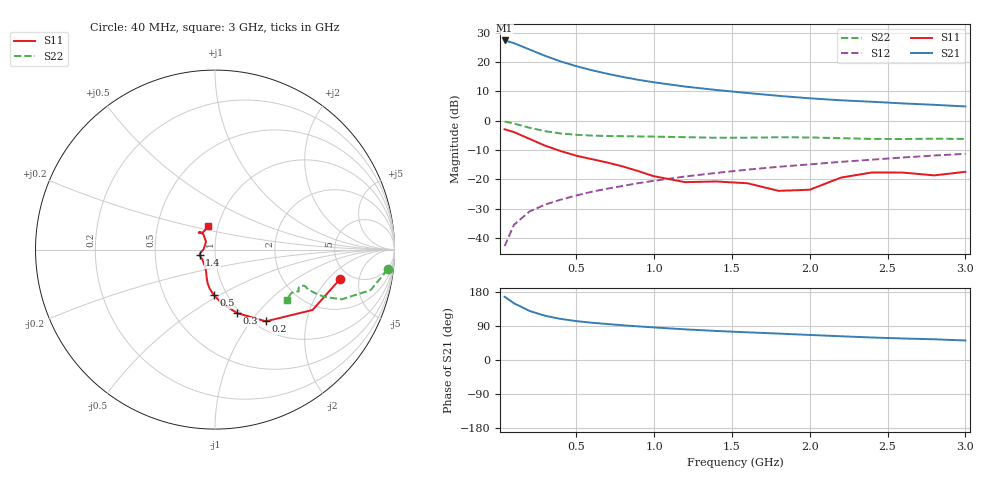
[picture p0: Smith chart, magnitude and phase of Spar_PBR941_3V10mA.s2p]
! Filename:  PBR941E.S2P  Version:  3.0
! NXP part #:  PBR941  Date: July 1998
! Bias condition:  Vce=3V, Ic=10mA
#  MHz  S  MA  R 50
! Freq  S11  S21  S12  S22
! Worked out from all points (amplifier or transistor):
!   21 points, 40 MHz to 3 GHz, reference 50 ohm
!   highest |S21| = 27.4 dB at 40 MHz (marker M1)
!   |S21| within 3 dB of that: start of sweep to 196 MHz
!   unconditionally stable (mu >= 1): 962.1 MHz to 2.337 GHz
!   at 300 MHz: K = 0.70, MSG = 25.4 dB, |S12| = -28.6 dB
!   at 1 GHz: K = 1.01, MAG = 16.3 dB, |S12| = -20.5 dB
!   at 3 GHz: K = 0.98, MSG = 8.1 dB, |S12| = -11.3 dB
!   S11 on the Smith chart (normalised r, x): 40 MHz: 4.05, -2.75; 200 MHz: 1.13, -1.19; 300 MHz: 0.96, -0.79; 500 MHz: 0.87, -0.47; 1.4 GHz: 0.84, -0.05; 3 GHz: 0.90, +0.24
40  0.714 -13.5  23.38 166.9  0.007242 83.1  0.9681 -6.6
100  0.6396 -31.7  21.03 149.8  0.01676 77.0  0.8963 -14.6
200  0.4902 -54.6  16.39 129.4  0.02825 69.8  0.7578 -21.5
300  0.3752 -70.7  12.78 116.7  0.03707 69.3  0.6625 -23.4
400  0.3033 -82.4  10.26 108.5  0.04498 70.3  0.6066 -23.5
500  0.2534 -91.6  8.526 102.7  0.05296 71.5  0.5748 -23.2
600  0.2208 -97.5  7.264 98.4  0.06143 73.0  0.5574 -22.8
700  0.1933 -102.2  6.318 94.8  0.06938 74.2  0.5489 -22.5
800  0.1657 -106.1  5.576 91.6  0.07722 74.9  0.5441 -22.2
900  0.1378 -110.9  4.984 88.7  0.08619 75.6  0.5402 -22.1
1000  0.1128 -118.3  4.518 85.9  0.09436 76.0  0.5357 -22.1
1200  0.08958 -141.9  3.82 80.8  0.1119 76.2  0.5233 -22.6
1400  0.09187 -159.6  3.344 76.6  0.1286 76.3  0.5126 -24.0
1600  0.08573 -165.4  2.97 73.0  0.1462 76.4  0.5139 -25.3
1800  0.06358 177.7  2.655 69.7  0.1636 76.7  0.5214 -26.2
2000  0.06646 138.7  2.412 66.1  0.18 76.0  0.5186 -26.8
2200  0.1068 127.1  2.23 62.6  0.1987 75.2  0.5032 -27.6
2400  0.131 131.3  2.104 59.4  0.2164 74.7  0.4892 -29.7
2600  0.1303 134.4  1.972 56.8  0.2359 74.3  0.4872 -32.5
2800  0.1167 125.3  1.866 54.6  0.2551 73.9  0.494 -34.3
3000  0.1344 105.7  1.751 51.5  0.272 72.8  0.4897 -34.9
